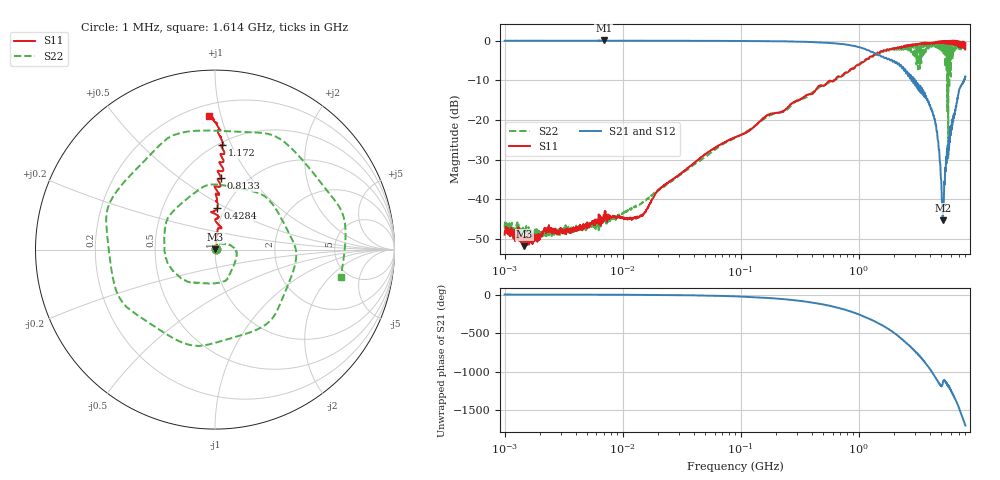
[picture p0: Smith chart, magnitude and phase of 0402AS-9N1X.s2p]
!s-Parameter Generated by FASTRON Sdn. Bhd.
!FASTRON P/N : 0402AS-9N1X
!Keysight Technologies: E5071C_MY46733604_B.14.02
!Date: Mon Dec 01 10:29:32 2025
!Version  :Rev00  Mon Dec 01 10:29:32 2025
!Data & Calibration Information:
!Freq  S11:SOLT2(ON)  S21:SOLT2(ON)  S12:SOLT2(ON)  S22:SOLT2(ON)
!PortZ  Port1:50+j0  Port2:50+j0
!When reading reference impedance value at option line is always used.
! Remarks : This data is being provided solely for informational purposes.
# Hz S dB R 50
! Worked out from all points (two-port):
!   1601 points, 1 MHz to 8 GHz, reference 50 ohm
!   highest |S21| = 0.03 dB at 6.912 MHz (marker M1); lowest = -45.3 dB at 5.136 GHz (marker M2)
!   |S21| within 3 dB of the highest: start of sweep to 1.327 GHz
!   lowest |S11| = -51.8 dB at 1.468 MHz (marker M3), VSWR 1.01, Z = 50.2 + j0.0647 ohm
!   |S11| at or under -10 dB: start of sweep to 621.7 MHz
!   |S22| runs from -50.5 to -0.2 dB; largest |S21 - S12| = 0.016
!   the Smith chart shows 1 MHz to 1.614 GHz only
!   S11 on the Smith chart (normalised r, x): 1 MHz: 1.01, +0.00; 428.4 MHz: 0.92, +0.46; 813.3 MHz: 0.77, +0.73; 1.172 GHz: 0.52, +0.92; 1.614 GHz: 0.28, +0.92
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1000000  -48.90 20.9  -0.05 -0.3  -0.02 -0.3  -47.10 22.0
1468277  -51.80 14.5  -0.05 -0.4  -0.04 -0.4  -46.90 -2.6
4479405  -47.10 37.0  -0.04 -1.2  -0.04 -1.2  -47.30 45.0
6911657  -43.90 22.7  0.03 -2.4  0.01 -2.4  -44.50 33.0
2.00676e7  -37.60 58.3  -0.05 -5.3  -0.05 -5.3  -37.70 69.6
8.994653e7  -24.30 87.8  -0.09 -23.6  -0.09 -23.6  -24.50 32.2
4.006501e8  -13.40 92.5  -0.36 -104.0  -0.35 -104.0  -13.20 -123.0
4.284291e8  -12.60 86.6  -0.41 -111.0  -0.40 -111.0  -12.50 -132.0
8.132836e8  -7.92 85.3  -1.07 150.0  -1.07 150.0  -7.79 35.2
1.171668e9  -4.69 86.2  -2.39 58.7  -2.38 58.6  -4.54 -150.0
1.411421e9  -3.32 88.5  -3.30 -0.2  -3.30 -0.2  -3.58 88.2
1.613809e9  -2.57 92.5  -4.08 -48.2  -4.09 -48.3  -2.89 -12.2
1.7949e9  -2.35 95.1  -4.56 -90.7  -4.56 -90.8  -2.52 -98.5
2.114474e9  -1.76 102.0  -5.73 -170.0  -5.72 -170.0  -2.13 96.0
2.296158e9  -1.61 103.0  -6.41 144.0  -6.40 144.0  -2.33 3.5
2.486897e9  -1.43 106.0  -7.49 98.2  -7.47 98.1  -2.40 -92.1
2.839031e9  -1.24 111.0  -9.63 23.1  -9.60 22.8  -0.90 111.0
3.244011e9  -1.00 122.0  -11.40 -75.1  -11.40 -75.4  -1.57 -80.4
3.649388e9  -0.71 126.0  -14.10 -167.0  -14.10 -167.0  -1.74 82.3
3.973689e9  -0.59 135.0  -16.30 121.0  -16.30 120.0  -1.76 -82.6
5.136407e9  -0.27 163.0  -45.30 -82.2  -45.40 -82.2  -2.17 40.9
8e9  -0.64 -102.0  -9.10 100.0  -9.13 100.0  -2.41 139.0
